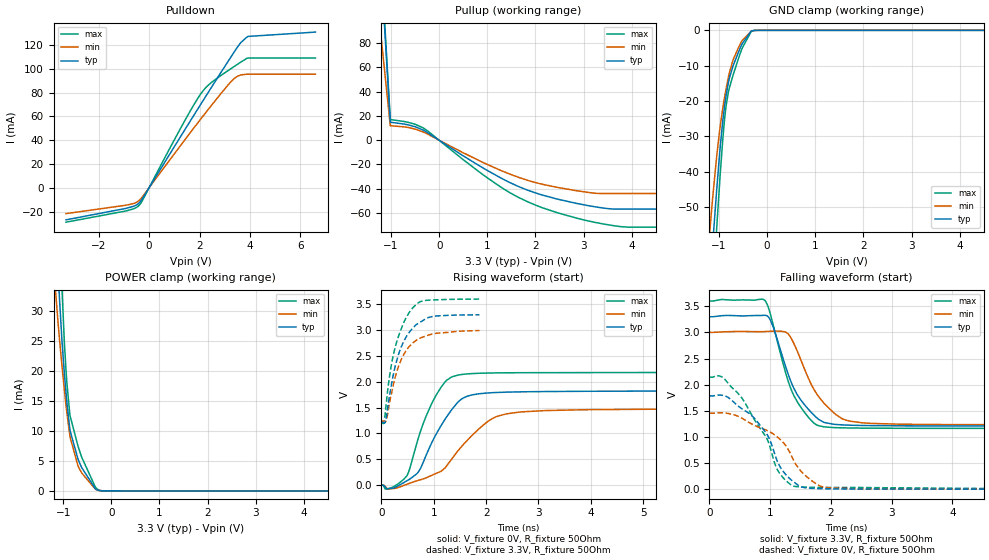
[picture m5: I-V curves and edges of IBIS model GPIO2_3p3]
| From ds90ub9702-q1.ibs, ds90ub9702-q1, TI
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|   GPIO2_3p3 Model
[Model]   GPIO2_3p3
Model_type   I/O
Polarity   Non-Inverting
Enable   Active-Low
Vinl = 0.8
Vinh = 2
Vmeas = 1.65
Vref = 0
Cref = 2pF
Rref = 100
|   typ   min   max
|   (nom PVT)   (fast PVT)   (slow PVT)
C_comp   5.699e-13   5.504e-13   6.225e-13
| Where nom  PVT is Nominal Process, 3.3V, 27C
|   Fast PVT is Strong Process,  3.6V, -40C
|   Slow PVT is Weak Process,   3V, 125C
[Voltage Range]   3.3   3   3.6
|Junction Temperature
[Temperature Range]   27   125   -40
[Pullup Reference]   3.3   3   3.6
[Pulldown Reference]   0   0   0
[Power Clamp Reference]   3.3   3   3.6
[GND Clamp Reference]   0   0   0
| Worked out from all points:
|   slope of the pulldown table from 0 to 0.495 V, typ, clamps not added: 29 ohm
|   slope of the pullup table from 0 to 0.495 V, typ, clamps not added: 38.9 ohm
|   GND clamp passes 1 mA (typ) near -0.37 V on its own axis
|   falling waveform, V_fixture 3.3V, R_fixture 50Ohm: 20-80 % time 444ps typ, 490ps min, 388ps max; typ from 3.3 V to 1.21 V
|   rising waveform, V_fixture 0V, R_fixture 50Ohm: 20-80 % time 565ps typ, 793ps min, 464ps max; typ from 0 V to 1.8 V
|   rising waveform, V_fixture 3.3V, R_fixture 50Ohm: 20-80 % time 342ps typ, 345ps min, 314ps max; typ from 1.21 V to 3.29 V
|   falling waveform, V_fixture 0V, R_fixture 50Ohm: 20-80 % time 530ps typ, 691ps min, 545ps max; typ from 1.79 V to 0 V
[Pulldown]
|   Voltage   I(typ)   I(min)   I(max)
-3.3V     -26.93mA   -21.7mA    -28.9mA
-888mV    -17.15mA   -14.52mA   -19.32mA
-620.4mV  -15.55mA   -13.2mA    -17.69mA
-416.4mV  -13.15mA   -11.02mA   -15.19mA
-243.6mV  -8.298mA   -6.901mA   -9.764mA
1.479V    50.9mA     42.06mA    58.86mA
2.057V    70.47mA    58.02mA    79.16mA
2.436V    83.19mA    68.27mA    87.87mA
3.303V    111.7mA    90.39mA    100.9mA
3.623V    121.6mA    94.78mA    105.4mA
3.871V    126.5mA    95.44mA    108.7mA
6.6V      130.8mA    95.44mA    109mA
[GND Clamp]
|   Voltage   I(typ)   I(min)   I(max)
-3.3V     -523.3mA   -450.4mA   -597.3mA
-1.3V     -93.64mA   -75.01mA   -113.5mA
-1.158V   -65.64mA   -51.56mA   -80.66mA
-1.128V   -59.9mA    -46.95mA   -73.84mA
-1.043V   -44.28mA   -35.01mA   -54.94mA
-920.4mV  -25.56mA   -21.98mA   -30.74mA
-861.3mV  -19.25mA   -17.2mA    -22.35mA
-805.2mV  -14.82mA   -13.3mA    -17.53mA
-709.5mV  -10.15mA   -8.452mA   -12.77mA
-573mV    -5.422mA   -4.221mA   -7.083mA
-330mV    -229.7uA   -220.5uA   -324.4uA
6.6V      0A         0A         0A
[Pullup]
|   Voltage   I(typ)   I(min)   I(max)
-3.3V     1.53A      889.5mA    1.586A
-1.016V   14.86mA    11.9mA     17.02mA
-636mV    12.54mA    10.4mA     14.62mA
-330mV    8.295mA    6.729mA    10.08mA
991.2mV   -24.75mA   -19.84mA   -30.76mA
1.461V    -34.78mA   -27.84mA   -43.1mA
1.866V    -41.6mA    -33.42mA   -51.23mA
2.436V    -48.34mA   -38.73mA   -59.52mA
3.079V    -53.8mA    -42.93mA   -66.37mA
3.513V    -56.41mA   -43.89mA   -69.71mA
3.752V    -56.73mA   -43.89mA   -71.13mA
6.6V      -56.73mA   -43.89mA   -71.65mA
[POWER Clamp]
|   Voltage   I(typ)   I(min)   I(max)
-3.3V     589.2mA    468.5mA    711.9mA
-1.158V   46.61mA    33.48mA    65.81mA
-1.079V   32.55mA    25.62mA    45.93mA
-1.025V   25.1mA     20.91mA    33.85mA
-940.5mV  16.39mA    14.33mA    20.13mA
-920.4mV  14.65mA    12.91mA    17.84mA
-855.6mV  10.05mA    8.972mA    12.53mA
-669.9mV  4.89mA     3.821mA    6.943mA
-330mV    350uA      291.5uA    617.1uA
-294mV    182.2uA    167.9uA    329.9uA
-111mV    8.274uA    10.02uA    10.1uA
6.6V      0A         0A         0A
[Ramp]
R_load = 50
|   typ   min   max
dV/dt_r   1.07753/5.6443e-10   0.880331/7.87651e-10   1.29184/4.62792e-10
dV/dt_f   1.2519/4.43338e-10   1.05704/4.85904e-10   1.43994/3.8782e-10
[Falling Waveform]
V_fixture = 3.3V
V_fixture_min = 3V
V_fixture_max = 3.6V
R_fixture = 50Ohm
|   Time   V(typ)   V(min)   V(max)
0s        3.3V       3V         3.6V
908ps     3.328V     3.015V     3.618V
1.019ns   3.197V     3.022V     3.285V
1.27ns    2.295V     2.996V     2.169V
1.392ns   1.928V     2.786V     1.788V
1.717ns   1.422V     1.92V      1.267V
2.046ns   1.243V     1.463V     1.179V
2.501ns   1.219V     1.272V     1.168V
3.848ns   1.21V      1.236V     1.164V
38.19ns   1.213V     1.236V     1.199V
[Rising Waveform]
V_fixture = 0V
V_fixture_min = 0V
V_fixture_max = 0V
R_fixture = 50Ohm
|   Time   V(typ)   V(min)   V(max)
0s        1.976uV    8.281uV    2.969uV
480.2ps   81.09mV    14.99mV    172.9mV
694.4ps   242.5mV    90.41mV    874.4mV
853.9ps   578mV      142.3mV    1.333V
1.237ns   1.307V     360.8mV    2.018V
1.545ns   1.673V     761.7mV    2.139V
2.035ns   1.781V     1.232V     2.166V
3.12ns    1.809V     1.441V     2.174V
7.647ns   1.82V      1.475V     2.177V
100ns     1.796V     1.467V     2.153V
[Rising Waveform]
V_fixture = 3.3V
V_fixture_min = 3V
V_fixture_max = 3.6V
R_fixture = 50Ohm
|   Time   V(typ)   V(min)   V(max)
0s        1.213V     1.238V     1.2V
48.01ps   1.203V     1.236V     1.199V
80.34ps   1.239V     1.228V     1.468V
154.1ps   1.724V     1.593V     2.103V
266.3ps   2.311V     2.1V       2.678V
409.8ps   2.743V     2.493V     3.1V
574.7ps   3.008V     2.725V     3.399V
734.7ps   3.144V     2.838V     3.541V
1.002ns   3.263V     2.927V     3.579V
1.874ns   3.292V     2.987V     3.595V
[Falling Waveform]
V_fixture = 0V
V_fixture_min = 0V
V_fixture_max = 0V
R_fixture = 50Ohm
|   Time   V(typ)   V(min)   V(max)
0s        1.786V     1.454V     2.144V
243.4ps   1.788V     1.46V      2.114V
519.5ps   1.551V     1.369V     1.768V
719.1ps   1.383V     1.234V     1.376V
965.3ps   1.017V     1.115V     919.4mV
1.141ns   477.2mV    976.1mV    329.7mV
1.392ns   135.7mV    540.1mV    57.01mV
1.646ns   19.01mV    197.1mV    36.52mV
1.94ns    6.171mV    28.57mV    33.55mV
5.649ns   156.4uV    187.4uV    3.515mV
